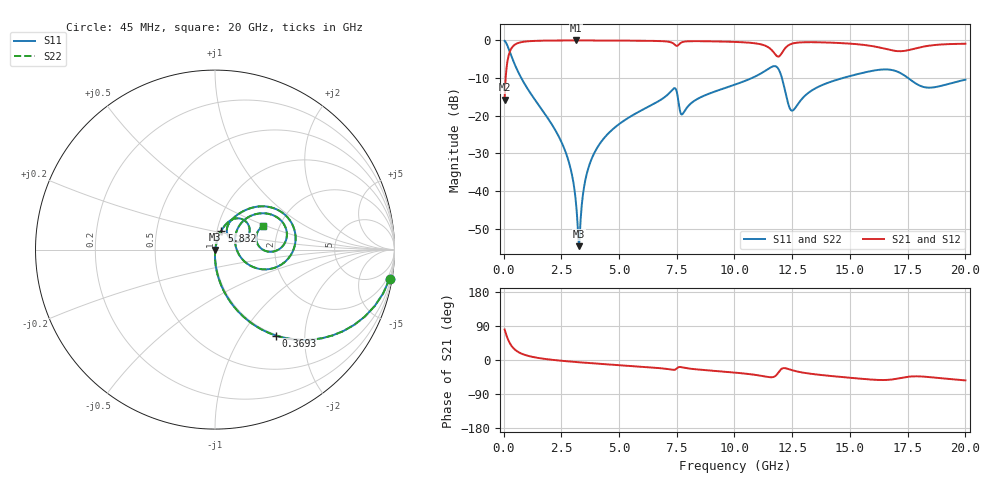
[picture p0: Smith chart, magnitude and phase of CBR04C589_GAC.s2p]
! S-parameter model data by Modelithics Inc.  support@modelithics.com 813-866-6335  Tampa FL USA
! S-Parameter data specifications:
! Substrate: 20-mil Rogers 4350B, substrate thickness, H=0.508mm, Dielectric constant, Er=3.75
! PCB Mounting Pad Footprint: Pad width, PadW=0.52mm , Pad length, PadL=0.52mm , Pad gap, PadG (edge-to-edge)=0.28mm , Reference planes=1.32mm apart
#  GHz  S  MA  R 50
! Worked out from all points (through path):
!   801 points, 45 MHz to 20 GHz, reference 50 ohm
!   highest |S21| = -0.02 dB at 3.138 GHz (marker M1); lowest = -15.7 dB at 45 MHz (marker M2)
!   group delay of S21, straight-line fit = 9.54 ps
!   lowest |S11| = -54.6 dB at 3.263 GHz (marker M3), VSWR 1.00, Z = 50.2 - j0.0253 ohm
!   |S11| at or under -10 dB: 768.7 MHz to 10.75 GHz (9.979 GHz wide, 173 % of centre); 12.06 GHz to 14.68 GHz (2.624 GHz wide, 19.6 % of centre); 17.52 GHz to end of sweep
!   |S22| runs from -54.6 to -0.1 dB; largest |S21 - S12| = 0
!   S11 on the Smith chart (normalised r, x): 45 MHz: 1, -12; 369.3 MHz: 0.98, -1.44; 5.832 GHz: 1.05, +0.23; 20 GHz: 1.65, +0.48
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0.045  0.9865 -9.5  0.1637 80.5  0.1637 80.5  0.9865 -9.5
0.369269  0.5868 -54.7  0.8091 35.3  0.8091 35.3  0.5868 -54.7
0.942975  0.2551 -76.7  0.9659 13.1  0.9659 13.1  0.2551 -76.7
2.564319  0.04097 -90.0  0.9974 -2.3  0.9974 -2.3  0.04097 -90.0
2.938475  0.01786 -88.7  0.998 -4.3  0.998 -4.3  0.01786 -88.7
3.138025  0.00691 -80.0  0.998 -5.3  0.998 -5.3  0.00691 -80.0
3.262744  0.001866 -7.8  0.998 -6.0  0.998 -6.0  0.001866 -7.8
3.387462  0.006602 66.7  0.998 -6.5  0.998 -6.5  0.006602 66.7
3.611956  0.01744 75.9  0.9978 -7.6  0.9978 -7.6  0.01744 75.9
4.036  0.03686 77.2  0.9971 -9.5  0.9971 -9.5  0.03686 77.2
5.83195  0.112 71.3  0.9903 -17.1  0.9903 -17.1  0.112 71.3
6.704981  0.1559 66.5  0.9811 -21.2  0.9811 -21.2  0.1559 66.5
7.403406  0.233 41.0  0.885 -25.9  0.885 -25.9  0.233 41.0
7.752619  0.1056 45.6  0.9509 -19.6  0.9509 -19.6  0.1056 45.6
10.0225  0.2593 54.3  0.9547 -33.3  0.9547 -33.3  0.2593 54.3
11.76856  0.4548 9.3  0.6516 -42.3  0.6516 -42.3  0.4548 9.3
12.06789  0.3065 -21.1  0.6932 -22.4  0.6932 -22.4  0.3065 -21.1
12.46699  0.1175 6.8  0.8991 -26.4  0.8991 -26.4  0.1175 6.8
13.36496  0.2185 45.5  0.9466 -36.8  0.9466 -36.8  0.2185 45.5
16.68248  0.4105 12.7  0.7537 -52.3  0.7537 -52.3  0.4105 12.7
18.30382  0.2373 9.0  0.8396 -44.4  0.8396 -44.4  0.2373 9.0
20  0.3013 26.3  0.9024 -53.8  0.9024 -53.8  0.3013 26.3
